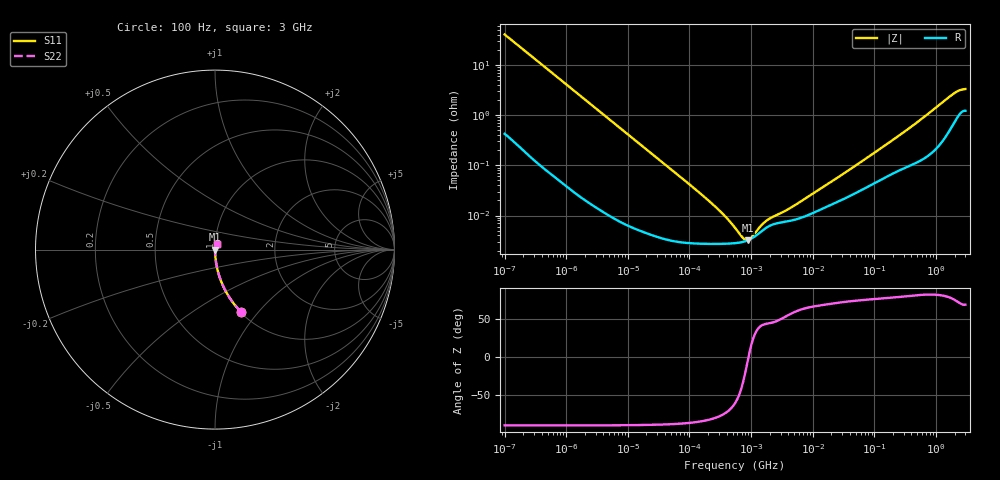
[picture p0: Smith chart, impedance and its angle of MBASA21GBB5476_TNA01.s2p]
! MBASA21GBB5476_TNA01  S-PARAMETER MODEL  ( Standard Model )
! Model Generated by TAIYO YUDEN Corporation (http://www.ty-top.com)
! Version 2.0
! TAIYO YUDEN Control No. 240306
! Copyright(c) 2012 TAIYO YUDEN CO.,LTD. All Rights Reserved.
! Product Description (link to TY-COMPAS)
! https://ds.yuden.co.jp/TYCOMPAS/or/detail?pn=MBASA21GBB5476MTNA01&u=M
! Products Name : Multilayer Ceramic Capacitors
! Characteristics :
!  Capacitance : 47 [uF] , Rated Voltage : 4 [V] , TCC : X5R
!  Case Size : 2.0 x 1.25 / 0.079 x 0.049 [mm/inch] , Thickness : 1.25 / 0.049 [mm/inch]
!  (Conditions: Temperature = 25 [degC] , DC Bias Voltage = 0 [V])
! External Node Assignments :
!  1  o---| |---o  2
! GND o---------o GND
! Frequency Range : 100Hz  -  3GHz  [ 401 STEP ]
# MHZ S RI R 50
! Freq[MHz].  S11 Real  S11 Imag  S21 Real  S21 Imag  S12 Real  S12 Imag  S22 Real  S22 Imag
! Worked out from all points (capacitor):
!   401 points, 100 Hz to 3 GHz, reference 50 ohm
!   read as one part in series: C = 39.2 uF near 109 Hz
!   lowest |Z| = 3.21 mohm at 879.4 kHz (marker M1)
!   series resonance near 907.6 kHz, so ESL is about 780 pH
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0.0001  0.1438 -0.3457  0.8562 0.3457  0.8562 0.3457  0.1438 -0.3457
0.000114  0.1154 -0.3144  0.8846 0.3144  0.8846 0.3144  0.1154 -0.3144
0.000175  0.0533 -0.2198  0.9467 0.2198  0.9467 0.2198  0.0533 -0.2198
0.000348  0.0146 -0.1155  0.9854 0.1155  0.9854 0.1155  0.0146 -0.1155
0.000724  0.00372 -0.0564  0.9963 0.0564  0.9963 0.0564  0.00372 -0.0564
0.001788  0.000754 -0.023  0.9992 0.023  0.9992 0.023  0.000754 -0.023
0.031977  3.82e-05 -0.00131  1 0.00131  1 0.00131  3.82e-05 -0.00131
0.150583  2.75e-05 -0.000272  1 0.000272  1 0.000272  2.75e-05 -0.000272
0.35615  2.73e-05 -0.000101  1 0.000101  1 0.000101  2.73e-05 -0.000101
0.405239  2.74e-05 -8.4e-05  1 8.4e-05  1 8.4e-05  2.74e-05 -8.4e-05
0.547723  2.81e-05 -4.96e-05  1 4.96e-05  1 4.96e-05  2.81e-05 -4.96e-05
0.87939  3.2e-05 -2.95e-06  1 2.95e-06  1 2.95e-06  3.2e-05 -2.95e-06
2.266852  6.64e-05 6.71e-05  0.9999 -6.71e-05  0.9999 -6.71e-05  6.64e-05 6.71e-05
2.579298  6.96e-05 7.42e-05  0.9999 -7.42e-05  0.9999 -7.42e-05  6.96e-05 7.42e-05
4.323298  7.85e-05 0.000117  0.9999 -0.000117  0.9999 -0.000117  7.85e-05 0.000117
9.794414  0.00011 0.000245  0.9999 -0.000245  0.9999 -0.000245  0.00011 0.000245
35.62563  0.000228 0.000716  0.9998 -0.000716  0.9998 -0.000716  0.000228 0.000716
175.1444  0.000638 0.0028  0.9994 -0.0028  0.9994 -0.0028  0.000638 0.0028
471.3361  0.00116 0.00678  0.9988 -0.00678  0.9988 -0.00678  0.00116 0.00678
1868.531  0.00688 0.0249  0.9931 -0.0249  0.9931 -0.0249  0.00688 0.0249
2419.119  0.0112 0.0289  0.9888 -0.0289  0.9888 -0.0289  0.0112 0.0289
3000  0.013 0.0301  0.987 -0.0301  0.987 -0.0301  0.013 0.0301
